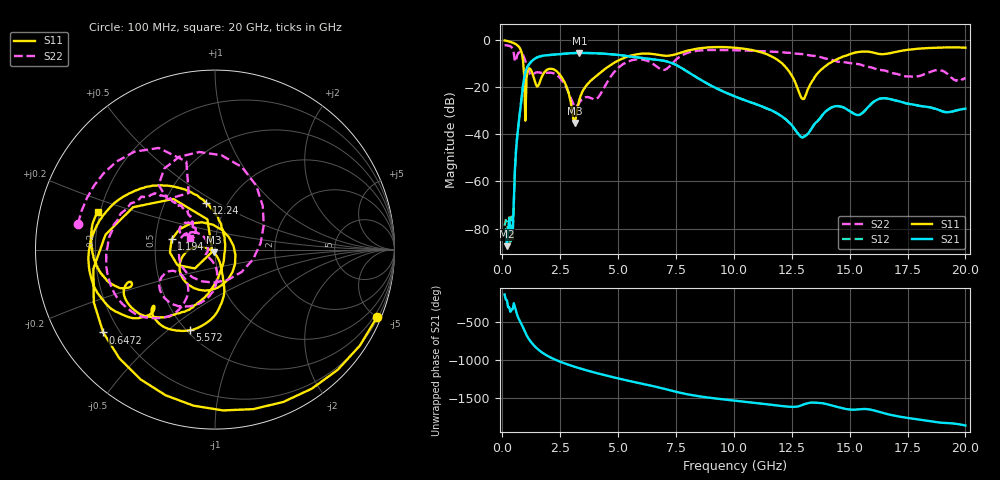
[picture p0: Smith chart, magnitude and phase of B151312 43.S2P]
!  2-Port S-parameters saved by WinCal
! VAR MeasName=S-Parameters (CALIBRATED_DATA) read from VNA (N5244A)
! VAR MeasDate=12/8/2015 5:47:17 PM
! VAR NAME=B151312 43
! VAR FILENAME=B151312 43.S2P
! VAR DATE=12/8/2015 5:47:17 PM
! VAR PHYS_PORTS=1,2
# Hz S DB R 50
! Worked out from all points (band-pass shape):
!   401 points, 100 MHz to 20 GHz, reference 50 ohm
!   highest |S21| = -5.50 dB at 3.334 GHz (marker M1); lowest = -87.4 dB at 199.5 MHz (marker M2)
!   |S21| within 3 dB of the highest: 1.324 GHz to 6.803 GHz (5.479 GHz wide, 135 % of centre)
!   lowest |S11| = -35.1 dB at 3.135 GHz (marker M3), VSWR 1.04, Z = 49.2 - j1.57 ohm
!   |S11| at or under -10 dB: 905.7 MHz to 4.778 GHz (3.873 GHz wide, 136 % of centre); 12.1 GHz to 14.11 GHz (2.014 GHz wide, 15.4 % of centre)
!   |S22| runs from -28.3 to -2.2 dB; largest |S21 - S12| = 0.0018
!   S11 on the Smith chart (normalised r, x): 100 MHz: 0.29, -4.99; 647.2 MHz: 0.14, -0.32; 1.194 GHz: 0.61, +0.07; 5.572 GHz: 0.52, -0.60; 12.24 GHz: 0.79, +0.44; 20 GHz: 0.19, +0.15
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1e8  -0.19 -22.6  -81.81 -145.9  -78.80 -163.5  -2.19 169.3
1.995e8  -0.38 -44.4  -87.43 140.4  -77.16 103.0  -2.28 158.2
3.985e8  -0.94 -87.2  -81.10 15.0  -74.90 -7.3  -3.02 129.5
6.4725e8  -2.21 -143.5  -40.60 -55.7  -40.66 -55.8  -6.41 131.1
9.955e8  -34.19 -140.9  -13.74 77.9  -13.74 77.9  -8.87 42.5
1.1945e9  -12.10 166.7  -9.80 -27.0  -9.80 -27.0  -14.26 -40.0
1.44325e9  -18.68 70.4  -7.68 -113.4  -7.68 -113.4  -13.81 -142.1
1.74175e9  -14.91 -65.4  -6.70 173.2  -6.70 173.3  -13.98 -177.9
2.289e9  -12.81 -149.3  -6.15 84.3  -6.15 84.3  -14.42 153.0
3.13475e9  -35.13 -114.8  -5.53 -9.5  -5.53 -9.5  -28.07 170.2
3.33375e9  -25.17 -70.3  -5.50 -28.2  -5.50 -28.2  -26.47 -161.0
3.43325e9  -22.47 -69.5  -5.50 -37.2  -5.50 -37.2  -25.17 -155.0
4.279e9  -13.49 -76.1  -5.74 -106.6  -5.74 -106.7  -22.25 -95.0
5.5725e9  -6.55 -107.4  -7.04 160.8  -7.04 160.8  -8.67 -121.1
6.7665e9  -6.32 -136.8  -8.46 81.4  -8.45 81.3  -11.95 -151.3
7.9605e9  -4.62 -139.4  -13.19 -5.2  -13.19 -5.4  -5.59 -133.5
1.005e10  -3.27 173.2  -23.95 -90.8  -23.95 -91.0  -4.35 -178.3
1.2239e10  -11.56 101.0  -33.59 -165.7  -33.61 -165.5  -5.37 153.4
1.29355e10  -24.78 13.2  -41.23 -149.1  -41.27 -149.0  -5.92 144.3
1.338325e10  -17.44 -78.6  -37.19 -114.8  -37.10 -115.2  -6.67 138.5
1.67165e10  -5.67 -156.2  -25.01 87.9  -24.90 87.3  -13.60 129.0
2e10  -3.27 162.2  -29.11 -53.9  -29.24 -54.3  -16.13 155.3
